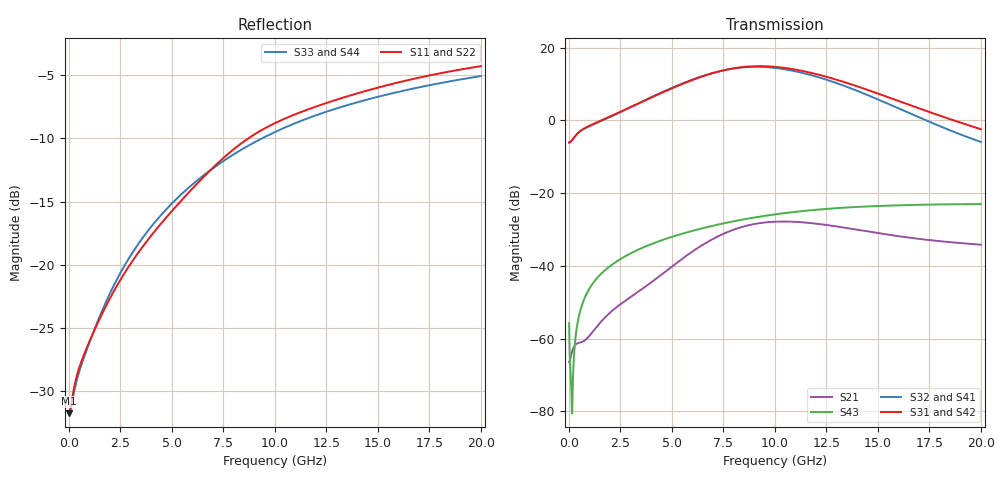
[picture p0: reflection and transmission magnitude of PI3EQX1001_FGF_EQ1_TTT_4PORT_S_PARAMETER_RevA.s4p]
! NPort=4 DATA=2000 NOISE=0 GROUPDELAY=0 COMPLEX_DATAFORMAT=POLAR
! NumOfBlock=1 NumOfParam=0
! .MODEL Smodel S TSTONEFILE=PI3EQX1001_FGF_EQ1_TTT_4PORT_S_PARAMETER_RevA.s4p TYPE=S
!  -- The above .MODEL line can be used for the S element in the netlist.
! The s parameter is extracted from the linear redriver, it is not bi-directional; only s(4,1)s(4,2) and s(3,1)s(3,2)
! should be the insertion loss
!Port definition:
!Port1 = input+
!Port2 = input¨C
!Port3 = output+
!Port4 = output-
# Hz S MA R  50
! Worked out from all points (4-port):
!   2000 points, 10 MHz to 20 GHz, reference 50 ohm
!   strongest paths, dB at 10 MHz, 5.01 GHz, 10.01 GHz, 15.01 GHz, 20 GHz:
!     S31: -6.1, 8.8, 14.7, 7.3, -2.4
!     S42: -6.1, 8.8, 14.7, 7.3, -2.5
!     S32: -6.1, 8.9, 14.4, 5.7, -5.9
!     S41: -6.1, 8.9, 14.4, 5.7, -6.0
!     S43: -55.8, -32.0, -25.9, -23.6, -23.0
!     S21: -66.4, -40.2, -27.9, -31.0, -34.2
!   lowest |S11| = -31.7 dB at 10 MHz (marker M1), VSWR 1.05, Z = 47.5 - j0.063 ohm
!   |S11| at or under -10 dB: start of sweep to 8.706 GHz
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1e7  0.02591 -178.5  0.0004922 2.7  3.669e-05 -0.2  4.787e-05 -0.1
     0.0004763 2.9  0.02597 -178.7  4.577e-05 -0.2  5.994e-05 -0.1
     0.4961 0.3  0.4961 -179.7  0.02616 178.4  0.001615 -59.2
     0.4958 -179.7  0.4959 0.3  0.001626 -58.9  0.02612 178.4
6.14e9  0.2061 -104.5  0.01608 100.6  2.314e-05 -30.7  3.302e-05 -29.1
        0.01675 99.0  0.2046 -104.5  3.027e-05 -26.5  4.198e-05 -24.4
        3.715 -48.6  3.755 134.4  0.2128 -111.1  0.03102 61.3
        3.742 134.4  3.711 -48.5  0.03101 61.2  0.2126 -111.1
8.26e9  0.2978 -107.1  0.03216 66.3  2.041e-05 -28.4  3.152e-05 -31.0
        0.03326 65.0  0.296 -107.1  2.938e-05 -25.8  3.931e-05 -24.6
        5.322 -109.0  5.279 74.2  0.2819 -113.4  0.04244 48.8
        5.253 74.2  5.32 -108.9  0.04233 48.6  0.2817 -113.4
1.028e10  0.3724 -112.9  0.03936 28.2  2.179e-05 -23.5  3.27e-05 -38.4
          0.04063 27.0  0.3697 -113.0  3.101e-05 -32.2  4.016e-05 -24.5
          5.338 -172.4  5.134 11.2  0.3433 -116.6  0.05239 35.5
          5.104 11.3  5.338 -172.3  0.05217 35.5  0.3431 -116.6
1.286e10  0.4463 -118.7  0.03416 -7.3  2.786e-05 -36.7  3.08e-05 -58.5
          0.03524 -8.4  0.4426 -118.7  2.915e-05 -50.7  4.503e-05 -34.4
          3.713 115.0  3.35 -60.4  0.4123 -120.9  0.06179 18.3
          3.328 -60.1  3.713 115.1  0.06163 18.4  0.4122 -120.9
1.547e10  0.5138 -123.4  0.026 -25.8  2.763e-05 -68.0  2.32e-05 -86.5
          0.02688 -26.8  0.5095 -123.4  2.126e-05 -75.4  4.225e-05 -55.9
          2.091 56.5  1.699 -116.2  0.4721 -125.0  0.0672 2.1
          1.687 -115.8  2.09 56.6  0.06715 2.2  0.4717 -124.9
2e10  0.6104 -131.1  0.01887 -36.9  1.343e-05 -152.0  1.1e-05 151.9
      0.01951 -38.5  0.605 -131.2  7.072e-06 135.5  1.613e-05 -94.9
      0.7551 -15.7  0.5047 -172.2  0.5577 -131.1  0.07053 -23.3
      0.5021 -171.3  0.754 -15.6  0.07051 -23.4  0.5576 -131.1
